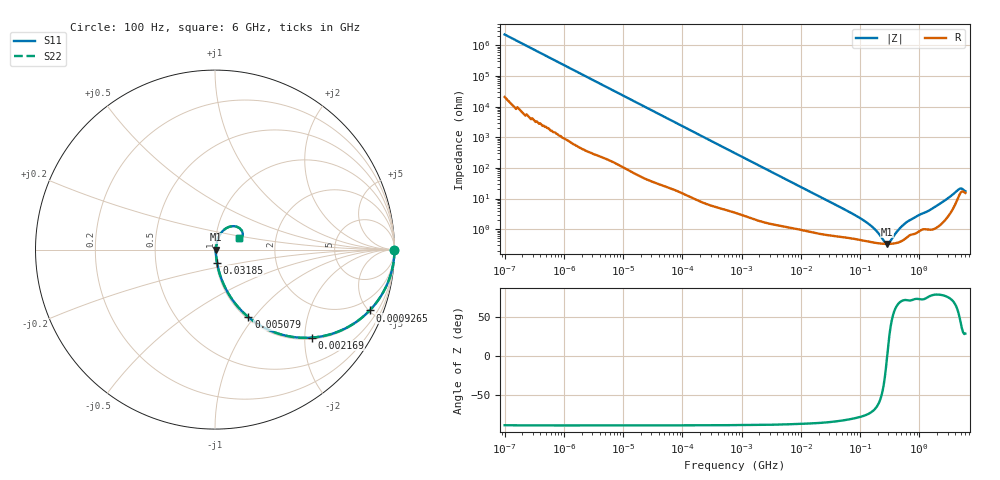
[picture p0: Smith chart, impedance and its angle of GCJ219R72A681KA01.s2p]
!Murata Part Number: GCJ219R72A681KA01
!These Parameters are Measured in Series Mode Connection
!Data Generated on Mar 13, 2026
!  o--ll--o
!Port1  Port2
!  o------o
!Operation Temp=25[degC], DC Bias Voltage=0[V]
!Freq. Start=100[Hz] Stop=6[GHz] 401[Steps]
# Hz S RI R 50
!Freq.(Hz) S11(Real) S11(Imag) S21(Real) S21(Imag) S12(Real) S12(Imag) S22(Real) S22(Imag)
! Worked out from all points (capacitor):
!   401 points, 100 Hz to 6 GHz, reference 50 ohm
!   read as one part in series: C = 696 pF near 109 Hz
!   lowest |Z| = 330 mohm at 285.7 MHz (marker M1)
!   series resonance near 287.2 MHz, so ESL is about 440 pH
!   S11 on the Smith chart (normalised r, x): 100 Hz: open; 926.5 kHz: 1.06, -5.07; 2.169 MHz: 1.04, -2.18; 5.079 MHz: 1.02, -0.93; 31.85 MHz: 1.01, -0.15; 6 GHz: 1.30, +0.17
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100  1 -4.38e-05  4e-07 4.38e-05  4e-07 4.38e-05  1 -4.38e-05
245  1 -0.000107  6e-07 0.000107  6e-07 0.000107  1 -0.000107
2008  1 -0.000874  4e-06 0.000874  4e-06 0.000874  1 -0.000874
40335  0.9996 -0.0174  0.000393 0.0174  0.000393 0.0174  0.9996 -0.0174
231233  0.9896 -0.0981  0.0104 0.0981  0.0104 0.0981  0.9896 -0.0981
774597  0.8989 -0.2959  0.1011 0.2959  0.1011 0.2959  0.8989 -0.2959
926525  0.8622 -0.3387  0.1378 0.3387  0.1378 0.3387  0.8622 -0.3387
2169299  0.5414 -0.4902  0.4586 0.4902  0.4586 0.4902  0.5414 -0.4902
5079039  0.1858 -0.376  0.8142 0.376  0.8142 0.376  0.1858 -0.376
8311524  0.0843 -0.2605  0.9157 0.2605  0.9157 0.2605  0.0843 -0.2605
1.555665e7  0.0307 -0.1489  0.9693 0.1489  0.9693 0.1489  0.0307 -0.1489
3.184506e7  0.0118 -0.0746  0.9882 0.0746  0.9882 0.0746  0.0118 -0.0746
1.334425e8  0.00421 -0.0153  0.9958 0.0153  0.9958 0.0153  0.00421 -0.0153
1.825626e8  0.00364 -0.00865  0.9964 0.00865  0.9964 0.00865  0.00364 -0.00865
2.61201e8  0.00331 -0.00178  0.9967 0.00178  0.9967 0.00178  0.00331 -0.00178
2.856706e8  0.00329 -9.72e-05  0.9967 9.72e-05  0.9967 9.72e-05  0.00329 -9.72e-05
3.124326e8  0.0033 0.0016  0.9967 -0.0016  0.9967 -0.0016  0.0033 0.0016
4.470121e8  0.00377 0.00882  0.9962 -0.00882  0.9962 -0.00882  0.00377 0.00882
6.395615e8  0.00597 0.0169  0.994 -0.0169  0.994 -0.0169  0.00597 0.0169
2.679998e9  0.0253 0.0804  0.9747 -0.0804  0.9747 -0.0804  0.0253 0.0804
4.586474e9  0.1198 0.1281  0.8802 -0.1281  0.8802 -0.1281  0.1198 0.1281
6e9  0.1364 0.0619  0.8636 -0.0619  0.8636 -0.0619  0.1364 0.0619
